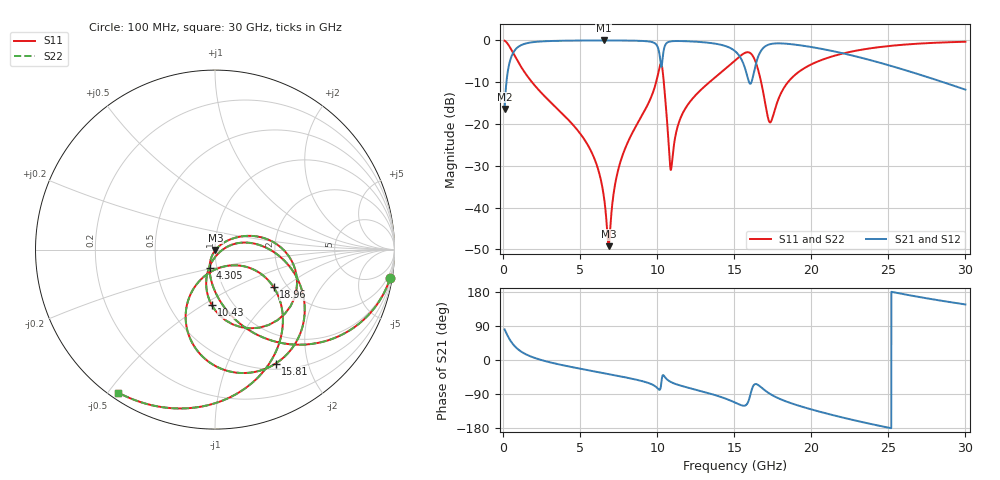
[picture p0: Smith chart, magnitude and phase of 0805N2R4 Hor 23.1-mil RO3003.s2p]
# GHz S MA R 50
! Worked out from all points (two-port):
!   3201 points, 100 MHz to 30 GHz, reference 50 ohm
!   highest |S21| = -0.03 dB at 6.519 GHz (marker M1); lowest = -16.4 dB at 100 MHz (marker M2)
!   |S21| within 3 dB of the highest: 648.4 MHz to 10.14 GHz (9.488 GHz wide, 176 % of centre); 16.66 GHz to 21.96 GHz (5.307 GHz wide, 27.5 % of centre)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
!   lowest |S11| = -49.2 dB at 6.846 GHz (marker M3), VSWR 1.01, Z = 50.3 - j0.223 ohm
!   |S11| at or under -10 dB: 1.876 GHz to 9.931 GHz (8.055 GHz wide, 136 % of centre); 10.43 GHz to 13.39 GHz (2.964 GHz wide, 24.9 % of centre); 16.75 GHz to 18.49 GHz (1.741 GHz wide, 9.88 % of centre)
!   |S22| runs from -49.2 to -0.1 dB; largest |S21 - S12| = 0
!   S11 on the Smith chart (normalised r, x): 100 MHz: 1, -12; 4.305 GHz: 0.92, -0.19; 10.43 GHz: 0.80, -0.55; 15.81 GHz: 0.57, -1.51; 18.96 GHz: 1.71, -0.84; 30 GHz: 0.02, -0.53
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0.1  0.9885 -9.2  0.1512 80.7  0.1512 80.7  0.9885 -9.2
0.5391563  0.7703 -42.6  0.6371 47.4  0.6371 47.4  0.7703 -42.6
1.398781  0.415 -73.1  0.9086 16.8  0.9086 16.8  0.415 -73.1
4.304688  0.1087 -106.2  0.9916 -17.4  0.9916 -17.4  0.1087 -106.2
5.089563  0.07309 -111.6  0.9945 -23.7  0.9945 -23.7  0.07309 -111.6
6.00525  0.03531 -115.8  0.9962 -30.7  0.9962 -30.7  0.03531 -115.8
6.519156  0.0144 -111.6  0.9964 -34.6  0.9964 -34.6  0.0144 -111.6
6.846188  0.003456 -40.0  0.9963 -37.2  0.9963 -37.2  0.003456 -40.0
7.640406  0.03653 40.2  0.995 -43.4  0.995 -43.4  0.03653 40.2
10.06978  0.4068 -4.1  0.7983 -76.5  0.7983 -76.5  0.4068 -4.1
10.43419  0.3108 -93.2  0.7774 -41.3  0.7774 -41.3  0.3108 -93.2
10.92006  0.02976 -27.6  0.974 -58.8  0.974 -58.8  0.02976 -27.6
11.89181  0.1599 14.1  0.9755 -71.8  0.9755 -71.8  0.1599 14.1
15.05  0.5743 -30.0  0.7436 -112.2  0.7436 -112.2  0.5743 -30.0
15.80684  0.7192 -61.9  0.3965 -117.3  0.3965 -117.3  0.7192 -61.9
16.0965  0.6904 -81.6  0.3092 -83.9  0.3092 -83.9  0.6904 -81.6
16.50763  0.4731 -109.1  0.6045 -64.8  0.6045 -64.8  0.4731 -109.1
17.32053  0.1043 -73.5  0.8987 -89.4  0.8987 -89.4  0.1043 -73.5
18.95569  0.3879 -32.6  0.8878 -117.6  0.8878 -117.6  0.3879 -32.6
20.03956  0.5198 -43.5  0.8293 -130.8  0.8293 -130.8  0.5198 -43.5
25.01978  0.8542 -89.6  0.5039 -178.6  0.5039 -178.6  0.8542 -89.6
30  0.962 -124.1  0.2573 146.6  0.2573 146.6  0.962 -124.1
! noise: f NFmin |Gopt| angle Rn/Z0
0.1  0.0009505  0.9372  1.382  0.003374
3.417  0.006327  0.7047  19.38  0.004089
6.743  0.01139  0.6861  36.64  0.006372
10.06  0.08747  0.932  53.56  0.2282
13.39  0.03446  0.7935  69.26  0.02348
16.7  0.1646  0.9431  85.05  0.3519
20.03  0.05442  0.8129  98.7  0.02613
23.35  0.05569  0.7962  111.3  0.01851
26.67  0.06781  0.8154  123.5  0.01779
30  0.08949  0.8491  135.8  0.01856
